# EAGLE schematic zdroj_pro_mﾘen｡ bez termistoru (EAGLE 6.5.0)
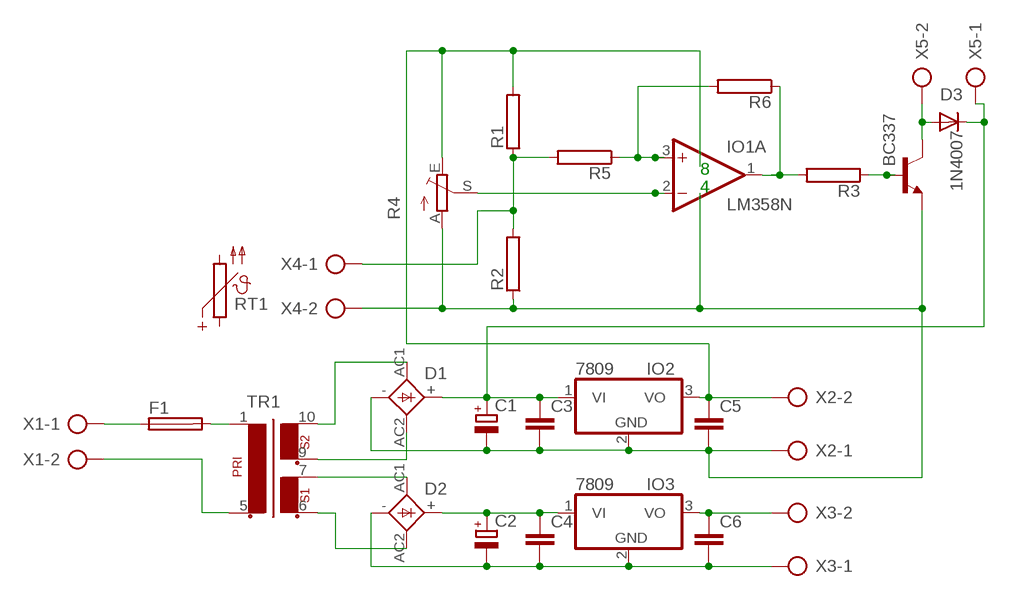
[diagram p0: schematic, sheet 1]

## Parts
C1  E5-10  [E5-10]
C2  E5-10  [E5-10]
C3  CK  [C3X5]
C4  CK  [C3X5]
C5  CK  [C3X5]
C6  CK  [C3X5]
D1  B250C1500  [WOM]
D2  B250C1500  [WOM]
D3  1N4007  [DO41-10]
F1  SH25  [SH25]
IO1  LM358N  [DIL08]
IO2  7809  7812TV  [TO220V]
IO3  7809  7812TV  [TO220V]
Q1  BC337  [TO92]
R1  0207/7  [0207/7]
R2  0207/7  [0207/7]
R3  0207/7  [0207/7]
R4  PT10V  [PT10V]
R5  0207/7  [0207/7]
R6  0207/7  [0207/7]
RT1  KTY-TO92  [TO92]
TR1  TRHEI422-2X12  [EI42-2B]
X1  AK500/2  [AK500/2]
X2  AK500/2  [AK500/2]
X3  AK500/2  [AK500/2]
X4  AK500/2  [AK500/2]
X5  AK500/2  [AK500/2]

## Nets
N$1: F1.1 X1.1
N$2: F1.2 TR1.1
N$3: D1.AC1 TR1.10
N$4: D1.AC2 TR1.9
N$5: D2.AC1 TR1.7
N$6: D2.AC2 TR1.6
N$7: C1.+ C3.1 D1.+ D3.C IO2.1(VI) X5.1
N$10: C2.+ C4.1 D2.+ IO3.1(VI)
N$11: C6.1 IO3.3(VO) X3.2
N$13: TR1.5 X1.2
N$14: D3.A Q1.3(C) X5.2
N$15: R1.1 R2.2 R5.2 X4.1
N$16: IO1.2(A:-IN) R4.S
N$17: Q1.2(B) R3.1
N$18: IO1.1(A:OUT) R3.2 R6.1
N$19: IO1.3(A:+IN) R5.1 R6.2
N$20: C2.- C4.2 C6.2 D2.- IO3.2(GND) X3.1
V+: C5.1 IO2.3(VO) R1.2 R4.E X2.2
V-: C1.- C3.2 C5.2 D1.- IO2.2(GND) Q1.1(E) R2.1 R4.A X2.1 X4.2
Unconnected: IO1.5(B:+IN) IO1.6(B:-IN) IO1.7(B:OUT) RT1.1 RT1.2

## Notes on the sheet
- 8
- 4

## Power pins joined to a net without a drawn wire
V+: IO1.8(P:V+)
V-: IO1.4(P:V-)

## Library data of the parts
C1 C2 = elektrolyticke kondenzatory radialni:E5: Elektrolytické kondenzátory radiální RM5,0
C3-C6 = kondenzatory:CK: Keramické kondenzátory rady CK
D1 D2 = diodove mustky a diaky:B250C1500: Diodový mustek
D3 = diody:1N4007: Usmernovací dioda
F1 = pojistky:SH25: FUSE HOLDER; MF: SCHURTER; MPN: 0031.8211; OC_FARNELL: 1162741; OC_NEWARK: 96B9380
IO1 = IO linear:LM358: OP AMP also LM158; LM258; LM2904 Source: http://cache.national.com/ds/LM/LM158.pdf
IO2 IO3 = linear:78*: Positive VOLTAGE REGULATOR Source: http://cache.national.com/ds/LM/LM78L05.pdf http://www.fairchildsemi.com/ds/LM/LM7805.pdf
Q1 = tranzistory NPN:BC337*: NPN Transistor
R1-R3 R5 R6 = rezistory:0207/*: Rezistor - vel. 0207
R4 = odporove trimry:PT10: Odporové trimry uhlíkové PT10
RT1 = termistory:KTY: Odporová teplotní cidla KTY
TR1 = transformatory:TRHEI422-2X12: Transformátor 2x12V
X1-X5 = Konektory:AK500/2: CONNECTOR; OC_FARNELL: unknown; OC_NEWARK: unknown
